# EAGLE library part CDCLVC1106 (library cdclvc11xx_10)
CDCLVC1106 3.3V and 2.5V LVCMOS High-Performance Clock Buffer - 1:6 Fan-out Source: http://www.ti.com/lit/ds/symlink/cdclvc1106.pdf
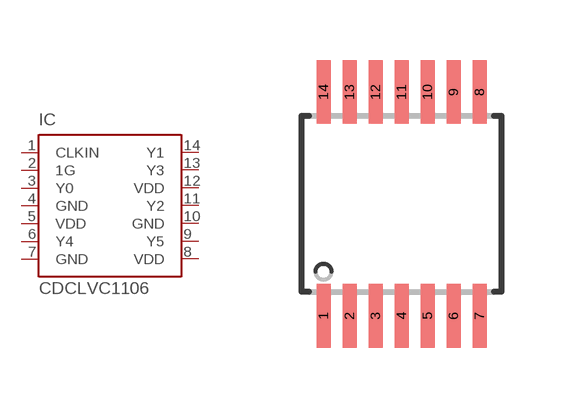
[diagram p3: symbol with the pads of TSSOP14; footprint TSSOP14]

Designator prefix IC

## CDCLVC1106PW (MF: Texas Instruments; MPN: CDCLVC1106; OC_FARNELL: 1829682; OC_NEWARK: 79R7912)  [TSSOP14]
1  CLKIN  in
2  1G  in
3  Y0  out
4  GND  pwr
5  VDD  pwr
6  Y4  out
7  GND  pwr
8  VDD  pwr
9  Y5  out
10  GND  pwr
11  Y2  out
12  VDD  pwr
13  Y3  out
14  Y1  out

## Footprint TSSOP14 (pad centres in mm)
TSSOP-14 Plastic Thin Srink Small Outline (PW) Source: http://www.ti.com/lit/ds/symlink/cdclvc1106.pdf
smd 0.35 x 1.6: 1 -1.95,-2.8; 2 -1.3,-2.8; 3 -0.65,-2.8; 4 0,-2.8; 5 0.65,-2.8; 6 1.3,-2.8; 7 1.95,-2.8; 8 1.95,2.8; 9 1.3,2.8; 10 0.65,2.8; 11 0,2.8; 12 -0.65,2.8; 13 -1.3,2.8; 14 -1.95,2.8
